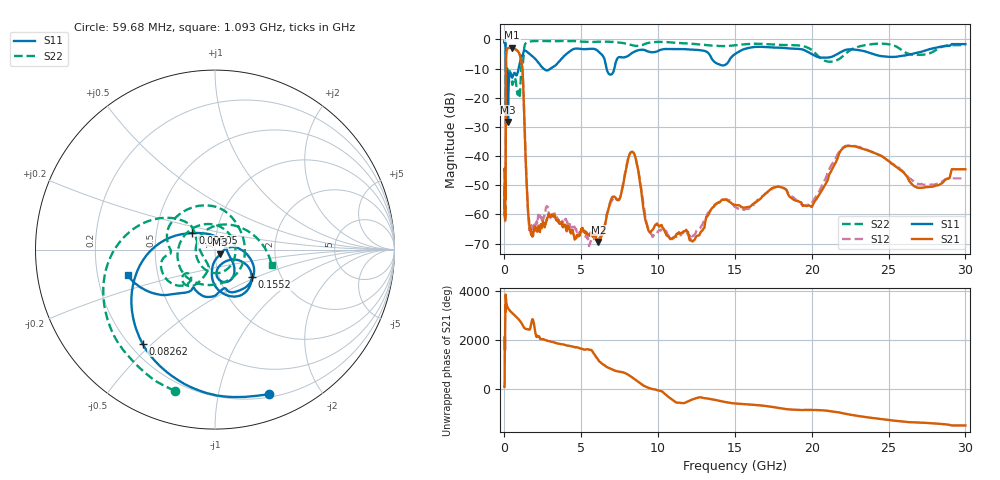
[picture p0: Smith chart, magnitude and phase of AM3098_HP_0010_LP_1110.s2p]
! Date/Time: Thu, Feb 28, 2019 8:33 AM
! Network Analyzer: Agilent Technologies E8364B Rev: A.07.50.67
! Sweep from 0.010 to 30.000 GHz, 1601 Points, Sweep Type: LOG
! Power Supply: 5.023 V, 0.002 A
# Hz S DB R 50
!freq MagS11 AngS11 MagS21 AngS21 MagS12 AngS12 MagS22 AngS22
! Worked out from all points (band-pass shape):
!   1601 points, 10 MHz to 30 GHz, reference 50 ohm
!   highest |S21| = -2.78 dB at 495.6 MHz (marker M1); lowest = -69.4 dB at 6.11 GHz (marker M2)
!   |S21| within 3 dB of the highest: 107.5 MHz to 1.028 GHz (920.5 MHz wide, 162 % of centre)
!   lowest |S11| = -28.3 dB at 232.8 MHz (marker M3), VSWR 1.08, Z = 52.8 - j2.75 ohm
!   |S11| at or under -10 dB: 92.14 MHz to 922.3 MHz (830.2 MHz wide, 164 % of centre); 2.533 GHz to 2.997 GHz (464.3 MHz wide, 16.8 % of centre); 6.646 GHz to 7.149 GHz (502.6 MHz wide, 7.29 % of centre)
!   |S22| runs from -22.4 to -0.5 dB; largest |S21 - S12| = 0.01
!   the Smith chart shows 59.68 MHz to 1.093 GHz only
!   S11 on the Smith chart (normalised r, x): 59.68 MHz: 0.23, -1.42; 82.62 MHz: 0.25, -0.47; 95.05 MHz: 0.76, +0.14; 155.2 MHz: 1.42, -0.47; 1.093 GHz: 0.33, -0.13
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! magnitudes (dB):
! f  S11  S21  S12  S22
! 10 MHz  -0.3  -44.9  -45.2  -0.6
! 38.04 MHz  -0.5  -60.7  -59.9  -1.0
! 59.68 MHz  -1.3  -50.4  -52.3  -1.8
! 72.91 MHz  -2.1  -54.8  -51.3  -2.5
! 82.62 MHz  -3.6  -35.8  -35.3  -4.0
! 95.05 MHz  -16.1  -12.2  -12.2  -20.1
! 144.7 MHz  -15.0  -3.5  -3.5  -12.9
! 155.2 MHz  -11.8  -3.5  -3.4  -11.1
! 232.8 MHz  -28.3  -2.9  -2.9  -12.0
! 495.6 MHz  -13.1  -2.8  -2.8  -15.3
! 550.5 MHz  -12.5  -3.0  -2.9  -15.1
! 1.093 GHz  -5.9  -7.4  -7.4  -9.7
! 1.582 GHz  -4.7  -61.3  -63.2  -0.8
! 2.084 GHz  -7.1  -65.2  -62.9  -0.5
! 6.11 GHz  -4.1  -69.4  -68.0  -0.8
! 7.926 GHz  -5.9  -44.0  -43.5  -1.5
! 8.501 GHz  -4.1  -40.1  -40.1  -2.2
! 9.586 GHz  -4.4  -65.6  -66.9  -1.0
! 12.37 GHz  -3.5  -68.7  -67.0  -1.5
! 19.9 GHz  -4.7  -57.1  -56.6  -3.3
! 22.56 GHz  -3.4  -36.6  -36.4  -3.5
! 30 GHz  -1.6  -44.5  -47.7  -1.9
